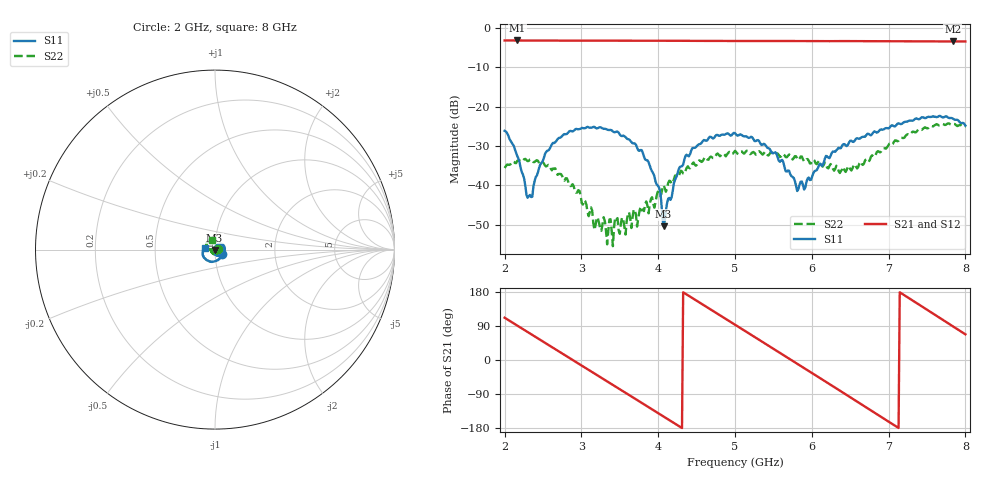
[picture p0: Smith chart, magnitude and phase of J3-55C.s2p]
!Agilent Technologies,E8364B,MY43040699,A.07.50.67
!Agilent E8364B: A.07.50.67
!Date: Friday, June 06, 2025 09:14:54
!Correction: S11(Full 2 Port(1,2))
!S21(Full 2 Port(1,2))
!S12(Full 2 Port(1,2))
!S22(Full 2 Port(1,2))
!S2P File: Measurements: S11, S21, S12, S22:
# Hz S  dB  R 50
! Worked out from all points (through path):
!   401 points, 2 GHz to 8 GHz, reference 50 ohm
!   highest |S21| = -3.17 dB at 2.165 GHz (marker M1); lowest = -3.4 dB at 7.835 GHz (marker M2)
!   group delay of S21, straight-line fit = 353 ps
!   lowest |S11| = -50.4 dB at 4.07 GHz (marker M3), VSWR 1.01, Z = 49.7 - j0.154 ohm
!   |S11| at or under -10 dB: start of sweep to end of sweep
!   |S22| runs from -55.5 to -24.2 dB; largest |S21 - S12| = 0.003
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2e9  -26.12 -33.1  -3.18 111.6  -3.18 111.6  -35.57 10.7
2.165e9  -32.55 -43.5  -3.17 90.8  -3.19 90.8  -33.74 -14.5
2.33e9  -42.43 15.8  -3.19 70.0  -3.19 70.0  -33.44 -37.1
2.6e9  -30.20 63.8  -3.20 36.0  -3.21 36.1  -35.70 -77.9
3.005e9  -25.38 24.5  -3.22 -14.9  -3.23 -14.9  -44.53 -141.8
3.185e9  -25.38 4.1  -3.22 -37.5  -3.24 -37.5  -50.03 -166.0
3.38e9  -25.92 -16.5  -3.23 -62.1  -3.25 -62.1  -48.59 97.9
3.785e9  -31.04 -64.9  -3.24 -113.1  -3.26 -113.1  -46.36 57.6
4.01e9  -40.55 -109.7  -3.24 -141.6  -3.26 -141.5  -42.32 62.9
4.07e9  -50.38 -149.3  -3.25 -149.1  -3.26 -149.0  -39.99 72.2
4.265e9  -36.00 85.5  -3.26 -173.8  -3.28 -173.7  -37.78 59.4
4.46e9  -30.47 50.1  -3.27 161.5  -3.29 161.7  -34.17 36.8
5e9  -26.73 -22.9  -3.31 93.2  -3.31 93.4  -31.21 -31.7
5.255e9  -28.74 -56.9  -3.31 60.8  -3.32 61.0  -31.76 -72.8
5.555e9  -32.88 -109.1  -3.31 22.6  -3.32 22.8  -31.88 -115.4
5.81e9  -41.44 179.4  -3.32 -9.9  -3.33 -9.7  -33.23 -154.6
6.005e9  -37.73 92.9  -3.33 -34.8  -3.34 -34.7  -33.79 -169.2
6.5e9  -28.66 3.1  -3.34 -98.2  -3.36 -98.1  -35.82 173.4
7.01e9  -25.38 -59.9  -3.39 -163.9  -3.39 -163.8  -29.42 178.8
7.385e9  -23.17 -109.0  -3.41 147.7  -3.41 147.7  -25.86 159.5
7.835e9  -22.98 -166.5  -3.43 89.2  -3.42 89.3  -24.49 124.7
8e9  -24.80 170.5  -3.42 67.7  -3.41 67.8  -25.05 108.7
